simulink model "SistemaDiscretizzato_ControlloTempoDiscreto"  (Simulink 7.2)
settings: Solver=ode3  StartTime=0.0  StopTime=10.0  FixedStep=Ts  RelTol=1e-3
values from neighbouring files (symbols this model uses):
  X0 = [0.5 2 -0.5]'    [TSC130625ProvaMatlab.m]
undefined symbols (not defined in the file or in its folder): Az, Bz, Cz, K
libraries: simulink x1

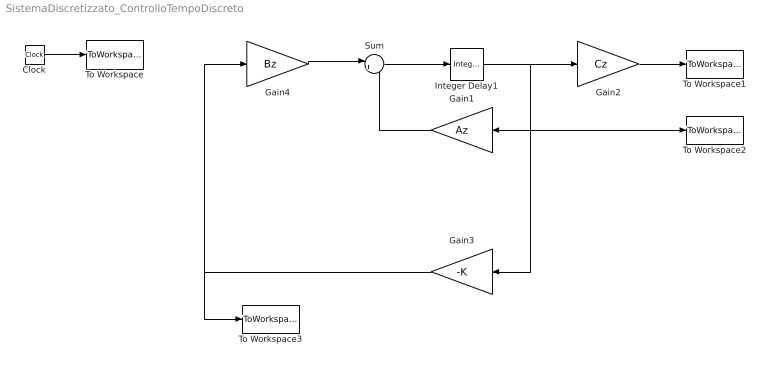
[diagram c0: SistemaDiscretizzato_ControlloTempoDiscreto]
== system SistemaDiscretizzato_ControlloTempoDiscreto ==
  Clock : Clock
  Gain1 : Gain  Orientation=left  Gain=Az  Multiplication=Matrix(K*u)  ParameterDataType=sfix(16)  ParameterScaling=2^0  OutDataType=sfix(16)  OutScaling=2^0
  Gain2 : Gain  Gain=Cz  Multiplication=Matrix(K*u)  ParameterDataType=sfix(16)  ParameterScaling=2^0  OutDataType=sfix(16)  OutScaling=2^0
  Gain3 : Gain  Orientation=left  Gain=-K  Multiplication=Matrix(K*u)  ParameterDataType=sfix(16)  ParameterScaling=2^0  OutDataType=sfix(16)  OutScaling=2^0
  Gain4 : Gain  Gain=Bz  Multiplication=Matrix(K*u)  ParameterDataType=sfix(16)  ParameterScaling=2^0  OutDataType=sfix(16)  OutScaling=2^0
  Integer Delay1 : simulink/Discrete/Integer Delay  vinit=X0  samptime=Ts  NumDelays=1
  Sum : Sum  Inputs=|++  OutDataType=sfix(16)  OutScaling=2^0
  To Workspace : ToWorkspace  VariableName=time  SampleTime=-1  SaveFormat=Array
  To Workspace1 : ToWorkspace  VariableName=y  SampleTime=-1  SaveFormat=Array
  To Workspace2 : ToWorkspace  VariableName=X  SampleTime=-1  SaveFormat=Array
  To Workspace3 : ToWorkspace  VariableName=ud  SampleTime=-1  SaveFormat=Array
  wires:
  Gain1/1 -> Sum/2
  Sum/1 -> Integer Delay1/1
  Integer Delay1/1 -> Gain2/1, Gain1/1, To Workspace2/1, Gain3/1
  Gain2/1 -> To Workspace1/1
  Gain4/1 -> Sum/1
  Gain3/1 -> Gain4/1, To Workspace3/1
  Clock/1 -> To Workspace/1
